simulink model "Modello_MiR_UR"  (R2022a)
settings: Solver=FixedStepAuto  StartTime=0.0  StopTime=time_s(end,1)  FixedStep=Sim.dt*10  RelTol=1e-3  EnableMultiTasking=on
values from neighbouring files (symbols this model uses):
  a = 0.250    (= 0.25)    [Modello_MiR_UR_script.m]    (also in Modello_MiR_2ruote_script.m; Modello_MiR_6ruote_script.m; Modello_MiR_6ruote_validato_script.m)
  a1 = 0.18265    [Modello_MiR_UR_script.m]    (also in UR_DHtable_e.m = 0; Modello_MiR_2ruote_script.m = deg2rad(5); Modello_MiR_6ruote_script.m = deg2rad(5); Modello_MiR_6ruote_validato_script.m)
  a2 = 0.40857    [Modello_MiR_UR_script.m]    (also in UR_DHtable_e.m = 612; Modello_MiR_2ruote_script.m = deg2rad(25); Modello_MiR_6ruote_script.m = deg2rad(25); Modello_MiR_6ruote_validato_script.m)
  Att_C1 = 0.01    [Modello_MiR_UR_script.m]    (also in Modello_MiR_6ruote_validato_script.m)
  Att_C2 = 0.01    [Modello_MiR_UR_script.m]    (also in Modello_MiR_6ruote_validato_script.m)
  Att_C5 = 0.01    [Modello_MiR_UR_script.m]    (also in Modello_MiR_6ruote_validato_script.m)
  Att_C6 = 0.01    [Modello_MiR_UR_script.m]    (also in Modello_MiR_6ruote_validato_script.m)
  b = 0.1875    [Modello_MiR_UR_script.m]    (also in Modello_MiR_2ruote_script.m; Modello_MiR_6ruote_script.m; Modello_MiR_6ruote_validato_script.m)
  b_caster = 0.07    [Modello_MiR_UR_script.m]    (also in Modello_MiR_2ruote_script.m; Modello_MiR_6ruote_script.m; Modello_MiR_6ruote_validato_script.m)
  bd = 0.205    [Modello_MiR_UR_script.m]    (also in Modello_MiR_2ruote_script.m; Modello_MiR_6ruote_script.m; Modello_MiR_6ruote_validato_script.m)
  F23MIR = @(u) (mv*9.801/4)-(mv*h*u(5)+(mv*9.801/4)*(2*a-b_caster*(cos(u(1))+cos(u(2)))))/(4*a-b_caster*(cos(u(1))+cos(u(2)))+b_caster*(cos(u(3))+cos(u(4))))    [Modello_MiR_UR_script.m]
  F23UR5 = @(u) (u(7)/4)-u(11)    [Modello_MiR_UR_script.m]
  F43MIR = @(u) (1/(2*bd))*(mv*u(6)*h+((mv*h*u(5)+(mv*9.801/4)*(2*a-b_caster*(cos(u(1))+cos(u(2)))))/(4*a-b_caster*(cos(u(1))+cos(u(2)))+b_caster*(cos(u(3))+cos(u(4)))))*(2*bd-b_caster*(sin(u(3))+sin(u(4))))+((mv*9.801/4)-(mv*h*u(5)+(mv*9.801/4)*(2*a-b_caster*(cos(u(1))+cos(u(2)))))/(4*a-b_caster*(cos(u(1))+cos(u(2)))+b_caster*(cos(u(3))+cos(u(4)))))*(2*bd-b_caster*(sin(u(1))+sin(u(2)))))    [Modello_MiR_UR_script.m]
  F43UR5 = @(u) (1/(2*bd))*(u(8) - u(6)*H +u(11)*(2*bd-b_caster*(sin(u(3))+sin(u(4))))+u(12)*(2*bd-b_caster*(sin(u(1))+sin(u(2)))))    [Modello_MiR_UR_script.m]
  F63MIR = @(u) (mv*h*u(5)+(mv*9.801/4)*(2*a-b_caster*(cos(u(1))+cos(u(2)))))/(4*a-b_caster*(cos(u(1))+cos(u(2)))+b_caster*(cos(u(3))+cos(u(4))))    [Modello_MiR_UR_script.m]
  F63UR5 = @(u)(-a*u(7)/2 -u(5)*H -u(9) +(u(7)/4)*(2*a-b_caster*(cos(u(1))+cos(u(2)))))/(4*a-b_caster*(cos(u(1))+cos(u(2)))+b_caster*(cos(u(3))+cos(u(4))))    [Modello_MiR_UR_script.m]
  f_c = 0.29564    [Modello_MiR_UR_script.m]    (also in Modello_MiR_6ruote_validato_script.m)
  f_d3 = 0.35846    [Modello_MiR_UR_script.m]    (also in Modello_MiR_6ruote_validato_script.m)
  f_d4 = 0.2333    [Modello_MiR_UR_script.m]    (also in Modello_MiR_6ruote_validato_script.m)
  fa_c = 0.27474    [Modello_MiR_UR_script.m]    (also in Modello_MiR_6ruote_validato_script.m)
  fa_d3 = 0.3694    [Modello_MiR_UR_script.m]    (also in Modello_MiR_6ruote_validato_script.m)
  fa_d4 = 0.28065    [Modello_MiR_UR_script.m]    (also in Modello_MiR_6ruote_validato_script.m)
  fm_fun = @(u) (u <= -am2 || u >= am2) * 0 + (u > -am2 && u <= -am1) * (- u* Mza/(am2 -am1) - Mza* am2/(am2 -am1)) +           + (u > -am1 && u <= am1) * (Mza * u / am1) + (u > am1 && u < am2) * (Mza * u /(am1 -am2) - Mza * am2 /(am1 - am2))    [Modello_MiR_UR_script.m]    (also in Modello_MiR_6ruote_script.m = @(u) (u <= -am2 | u >= am2)*0 + (u > -am2 && u <= -am1)*(- u; Modello_MiR_6ruote_validato_script.m)
  Hi = 1    [UR5e_data.m]
  Icw_1 = 1/2 * mcw * rc^2    (= 0.002004225735)    [Modello_MiR_UR_script.m]    (also in Modello_MiR_2ruote_script.m; Modello_MiR_6ruote_script.m; Modello_MiR_6ruote_validato_script.m)
  Icw_2 = 1/12 * mcw * ec^2 + 1/4 * mcw * rc^2    (= 0.00104098243873)    [Modello_MiR_UR_script.m]    (also in Modello_MiR_2ruote_script.m; Modello_MiR_6ruote_script.m; Modello_MiR_6ruote_validato_script.m)
  Idw_1 = 1/2 * mdw * rd^2    (= 0.00551836278784)    [Modello_MiR_UR_script.m]    (also in Modello_MiR_2ruote_script.m; Transfer_Function_Gol_Gcl.m = Inertia_vect(jj,1); Modello_MiR_6ruote_script.m; Modello_MiR_6ruote_validato_script.m)
  iMax = 20.7*1.1    (= 22.77)    [Modello_MiR_UR_script.m]    (also in Modello_MiR_2ruote_script.m; Modello_MiR_6ruote_script.m; Modello_MiR_6ruote_validato_script.m)
  Iv = mv * (l^2 + w^2)  / 12    (= 6.75343333333)    [Modello_MiR_UR_script.m]    (also in Modello_MiR_2ruote_script.m; Modello_MiR_6ruote_script.m; Modello_MiR_6ruote_validato_script.m = 8.95033333333)
  Kc = 0.15    [Modello_MiR_UR_script.m]    (also in Modello_MiR_2ruote_script.m; Modello_MiR_6ruote_script.m; Modello_MiR_6ruote_validato_script.m)
  Ki_i = 1    [Modello_MiR_UR_script.m]    (also in Modello_MiR_2ruote_script.m; Modello_MiR_6ruote_script.m; Modello_MiR_6ruote_validato_script.m)
  Ki_v = 1    [Modello_MiR_UR_script.m]    (also in Modello_MiR_2ruote_script.m; Modello_MiR_6ruote_script.m; Modello_MiR_6ruote_validato_script.m)
  kk = 0.00005    (= 5e-05)    [Modello_MiR_UR_script.m]    (also in Modello_MiR_2ruote_script.m; Modello_MiR_6ruote_script.m; Modello_MiR_6ruote_validato_script.m)
  Kp_i = 5    [Modello_MiR_UR_script.m]    (also in Modello_MiR_2ruote_script.m; Modello_MiR_6ruote_script.m; Modello_MiR_6ruote_validato_script.m)
  Kp_v = 5    [Modello_MiR_UR_script.m]    (also in Modello_MiR_2ruote_script.m; Modello_MiR_6ruote_script.m; Modello_MiR_6ruote_validato_script.m)
  kv = 1.5e-6    (= 1.5e-06)    [Modello_MiR_UR_script.m]    (also in Modello_MiR_2ruote_script.m; Modello_MiR_6ruote_script.m; Modello_MiR_6ruote_validato_script.m)
  L = R * tauE    (= 0.00181134822805)    [Modello_MiR_UR_script.m]    (also in Modello_MiR_2ruote_script.m; Modello_MiR_6ruote_script.m; Modello_MiR_6ruote_validato_script.m)
  mcw = rc^2 * pi * ec * rhopoliu + 1    (= 1.02616357632)    [Modello_MiR_UR_script.m]    (also in Modello_MiR_2ruote_script.m; Modello_MiR_6ruote_script.m; Modello_MiR_6ruote_validato_script.m)
  mv = 83    [Modello_MiR_UR_script.m]    (also in Modello_MiR_2ruote_script.m; Modello_MiR_6ruote_script.m; Modello_MiR_6ruote_validato_script.m = 110)
  Phi1_start = psi_mir(1,1)    [Modello_MiR_UR_script.m]    (also in Modello_MiR_6ruote_validato_script.m)
  Phi2_start = psi_mir(1,1)    [Modello_MiR_UR_script.m]    (also in Modello_MiR_6ruote_validato_script.m)
  Phi5_start = psi_mir(1,1)    [Modello_MiR_UR_script.m]    (also in Modello_MiR_6ruote_validato_script.m)
  Phi6_start = psi_mir(1,1)    [Modello_MiR_UR_script.m]    (also in Modello_MiR_6ruote_validato_script.m)
  Psi_start = psi_mir(1,1)    [Modello_MiR_UR_script.m]    (also in Modello_MiR_6ruote_script.m = 1.57079632679; Modello_MiR_6ruote_validato_script.m)
  q0 = [qset.q1.signals.values(1),qset.q2.signals.values(1),qset.q3.signals.values(1),qset.q4.signals.values(1),qset.q5.signals.values(1),qset.q6.signals.values(1)]    [UR5e_simmot.m]
  R = velMax * TorqueMax / (iMax)^2    (= 1.81134822805)    [Modello_MiR_UR_script.m]    (also in Modello_MiR_2ruote_script.m; Modello_MiR_6ruote_script.m; Modello_MiR_6ruote_validato_script.m)
  rap_rid = 10.167    [Modello_MiR_UR_script.m]    (also in Modello_MiR_2ruote_script.m; Modello_MiR_6ruote_script.m; Modello_MiR_6ruote_validato_script.m)
  rc = 0.125/2    (= 0.0625)    [Modello_MiR_UR_script.m]    (also in Modello_MiR_2ruote_script.m; Modello_MiR_6ruote_script.m; Modello_MiR_6ruote_validato_script.m)
  rd = 0.1    [Modello_MiR_UR_script.m]    (also in Modello_MiR_2ruote_script.m; Modello_MiR_6ruote_script.m; Modello_MiR_6ruote_validato_script.m)
  s = 1i*s    [Transfer_Function_Gol_Gcl.m]
  s1 = 0.18987    [Modello_MiR_UR_script.m]    (also in Modello_MiR_2ruote_script.m = 0.2; Modello_MiR_6ruote_script.m = 0.2; Modello_MiR_6ruote_validato_script.m)
  s2 = 0.99533    [Modello_MiR_UR_script.m]    (also in Modello_MiR_2ruote_script.m = 0.8; Modello_MiR_6ruote_script.m = 0.8; Modello_MiR_6ruote_validato_script.m)
  Sx = spline(x ,fl_fun(x),zx)    [Modello_MiR_6ruote_script.m]
  Sy = spline(x ,ft_fun(x),zy)    [Modello_MiR_6ruote_script.m]
  tau_i = 1/(2000*2*pi)    (= 7.95774715459e-05)    [UR5e_data.m]    (also in Transfer_Function_Gol_Gcl.m = Kp_i/Ki_i)
  VaMax = Kc * velMax    (= 41.2443991527)    [Modello_MiR_UR_script.m]    (also in Modello_MiR_2ruote_script.m; Modello_MiR_6ruote_script.m; Modello_MiR_6ruote_validato_script.m)
  X_start = traj(1,1)    [Modello_MiR_UR_script.m]    (also in Modello_MiR_2ruote_script.m = input('Inserire coordinata x iniziale'); Modello_MiR_6ruote_script.m = input('Inserire coordinata x iniziale'); Modello_MiR_6ruote_validato_script.m)
  Y_start = traj(1,2)    [Modello_MiR_UR_script.m]    (also in Modello_MiR_2ruote_script.m = input('Inserire coordinata y iniziale'); Modello_MiR_6ruote_script.m = input('Inserire coordinata y iniziale'); Modello_MiR_6ruote_validato_script.m)
undefined symbols (not defined in the file or in its folder): deg, Driver1, Driver2, Driver3, Driver4, Driver5, Driver6, Ground, J1, J2, J3, J4, J5, J6, kg, L1, L2, L3, L4, L5, L6, m, Motor, N, X, Y, z, Z
libraries: sm_lib x33, nesl_utility x30, slpidlib x10
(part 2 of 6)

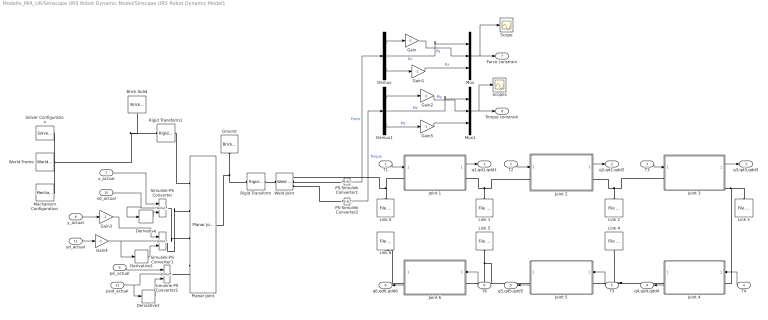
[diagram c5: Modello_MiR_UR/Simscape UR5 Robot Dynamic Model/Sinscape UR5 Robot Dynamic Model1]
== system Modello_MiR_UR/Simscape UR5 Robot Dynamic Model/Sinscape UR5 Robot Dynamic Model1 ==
  T1 : Inport
  T2 : Inport  Port=2
  T3 : Inport  Port=3
  T4 : Inport  Port=4
  T5 : Inport  Port=5
  T6 : Inport  Port=6
  x_actual : Inport  Port=7
  y_actual : Inport  Port=8
  psi_actual : Inport  Port=9
  xd_actual : Inport  Port=10
  yd_actual : Inport  Port=11
  psid_actual : Inport  Port=12
  Brick Solid : sm_lib/Body Elements/Brick Solid  GraphicAmbientColor=[0.15 0.15 0.15 1.0]  BasedOnType=Density  BrickDimensions=[100 100 1]  BrickDimensionUnits=m  CenterOfMass=[0 0 0]  CenterOfMassUnits=m  GraphicDiffuseColor=[0.5 0.5 0.5]  Density=1000  DensityUnits=kg/m^3  DoExposeReferenceFrame=on  GraphicEmissiveColor=[0.0 0.0 0.0 1.0]  ExportEntireGeometry=off  SerializedFrames=<Frames/>  MarkerShape=Sphere  MarkerSize=10  GraphicType=FromGeometry  InertiaType=CalculateFromGeometry  Mass=1  MassUnits=kg  MomentsOfInertia=[1 1 1]  MomentsOfInertiaUnits=kg*m^2  GraphicOpacity=1.0  ProductsOfInertia=[0 0 0]  ProductsOfInertiaUnits=kg*m^2  GraphicShininess=75  GraphicSpecularColor=[0.5 0.5 0.5 1.0]  GraphicVisPropType=SimpleVisualProperties
  Demux : Demux  Outputs=3
  Demux1 : Demux  Outputs=3
  Derivative : Derivative
  Derivative1 : Derivative
  Derivative2 : Derivative
  Gain{,1..5} (6 alike) : Gain  Gain=-1
  Ground : sm_lib/Body Elements/Brick Solid  GraphicAmbientColor=[0.15 0.15 0.15 1.0]  BasedOnType=Density  BrickDimensions=[Ground.l Ground.w Ground.h]  BrickDimensionUnits=m  CenterOfMass=[0 0 0]  CenterOfMassUnits=m  GraphicDiffuseColor=[1.0 1.0 1.0]  Density=1000  DensityUnits=kg/m^3  DoExposeReferenceFrame=on  GraphicEmissiveColor=[0.0 0.0 0.0 1.0]  ExportEntireGeometry=off  SerializedFrames=<Frames/>  MarkerShape=Sphere  MarkerSize=10  GraphicType=FromGeometry  InertiaType=CalculateFromGeometry  Mass=1  MassUnits=kg  MomentsOfInertia=[1 1 1]  MomentsOfInertiaUnits=kg*m^2  GraphicOpacity=1.0  ProductsOfInertia=[0 0 0]  ProductsOfInertiaUnits=kg*m^2  GraphicShininess=75  GraphicSpecularColor=[0.5 0.5 0.5 1.0]  GraphicVisPropType=SimpleVisualProperties
  Joint 1 : Subsystem
  Joint 2 : Subsystem
  Joint 3 : Subsystem
  Joint 4 : Subsystem
  Joint 5 : Subsystem
  Joint 6 : Subsystem
  Link 0 : sm_lib/Body Elements/File Solid  ExtGeomFileName=C:\Users\user\Desktop\Modello MiR-UR validato\GROUND.stp  UnitType=Custom  ExtGeomFileUnits=mm  StepReaderType=HEX  ExportConvexHullGeometry=off  InertiaType=Custom  Mass=1  MassUnits=kg  CenterOfMass=[0 0 0]  CenterOfMassUnits=m  MomentsOfInertia=[1 1 1]  MomentsOfInertiaUnits=kg*m^2  ProductsOfInertia=[0 0 0]  ProductsOfInertiaUnits=kg*m^2  BasedOnType=DensityFromFile  Density=1000  DensityUnits=kg/m^3  DoExposeReferenceFrame=on  SerializedFrames=<Frames/>  GraphicType=FromGeometry  MarkerShape=Sphere  MarkerSize=10  GraphicVisPropType=SimpleVisualProperties  GraphicDiffuseColor=[0.5 0.5 0.5]  GraphicSpecularColor=[0.5 0.5 0.5 1.0]  GraphicAmbientColor=[0.15 0.15 0.15 1.0]  GraphicEmissiveColor=[0.0 0.0 0.0 1.0]  GraphicShininess=75  GraphicOpacity=1.0
  Link 1 : sm_lib/Body Elements/File Solid  ExtGeomFileName=C:\Users\user\Desktop\Modello MiR-UR validato\UR5 old\LINK1.STEP  UnitType=Custom  ExtGeomFileUnits=mm  StepReaderType=HEX  ExportConvexHullGeometry=off  InertiaType=Custom  Mass=L1.Mass  MassUnits=kg  CenterOfMass=L1.CM  CenterOfMassUnits=m  MomentsOfInertia=L1.InertiaM  MomentsOfInertiaUnits=kg*m^2  ProductsOfInertia=L1.InertiaP  ProductsOfInertiaUnits=kg*m^2  BasedOnType=DensityFromFile  Density=1000  DensityUnits=kg/m^3  DoExposeReferenceFrame=on  SerializedFrames=<Frames/>  GraphicType=FromGeometry  MarkerShape=Sphere  MarkerSize=10  GraphicVisPropType=SimpleVisualProperties  GraphicDiffuseColor=[0.5 0.5 0.5]  GraphicSpecularColor=[0.5 0.5 0.5 1.0]  GraphicAmbientColor=[0.15 0.15 0.15 1.0]  GraphicEmissiveColor=[0.0 0.0 0.0 1.0]  GraphicShininess=75  GraphicOpacity=1.0
  Link 2 : sm_lib/Body Elements/File Solid  ExtGeomFileName=C:\Users\user\Desktop\Modello MiR-UR validato\UR5 old\LINK2.STEP  UnitType=Custom  ExtGeomFileUnits=mm  StepReaderType=HEX  ExportConvexHullGeometry=off  InertiaType=Custom  Mass=L2.Mass  MassUnits=kg  CenterOfMass=L2.CM  CenterOfMassUnits=m  MomentsOfInertia=L2.InertiaM  MomentsOfInertiaUnits=kg*m^2  ProductsOfInertia=L2.InertiaP  ProductsOfInertiaUnits=kg*m^2  BasedOnType=DensityFromFile  Density=1000  DensityUnits=kg/m^3  DoExposeReferenceFrame=on  SerializedFrames=<Frames/>  GraphicType=FromGeometry  MarkerShape=Sphere  MarkerSize=10  GraphicVisPropType=SimpleVisualProperties  GraphicDiffuseColor=[0.5 0.5 0.5]  GraphicSpecularColor=[0.5 0.5 0.5 1.0]  GraphicAmbientColor=[0.15 0.15 0.15 1.0]  GraphicEmissiveColor=[0.0 0.0 0.0 1.0]  GraphicShininess=75  GraphicOpacity=1.0
  Link 3 : sm_lib/Body Elements/File Solid  ExtGeomFileName=C:\Users\user\Desktop\Modello MiR-UR validato\UR5 old\LINK3.STEP  UnitType=Custom  ExtGeomFileUnits=mm  StepReaderType=HEX  ExportConvexHullGeometry=off  InertiaType=Custom  Mass=L3.Mass  MassUnits=kg  CenterOfMass=L3.CM  CenterOfMassUnits=m  MomentsOfInertia=L3.InertiaM  MomentsOfInertiaUnits=kg*m^2  ProductsOfInertia=L3.InertiaP  ProductsOfInertiaUnits=kg*m^2  BasedOnType=DensityFromFile  Density=1000  DensityUnits=kg/m^3  DoExposeReferenceFrame=on  SerializedFrames=<Frames/>  GraphicType=FromGeometry  MarkerShape=Sphere  MarkerSize=10  GraphicVisPropType=SimpleVisualProperties  GraphicDiffuseColor=[0.5 0.5 0.5]  GraphicSpecularColor=[0.5 0.5 0.5 1.0]  GraphicAmbientColor=[0.15 0.15 0.15 1.0]  GraphicEmissiveColor=[0.0 0.0 0.0 1.0]  GraphicShininess=75  GraphicOpacity=1.0
  Link 4 : sm_lib/Body Elements/File Solid  ExtGeomFileName=C:\Users\user\Desktop\Modello MiR-UR validato\UR5 old\LINK4.STEP  UnitType=Custom  ExtGeomFileUnits=mm  StepReaderType=HEX  ExportConvexHullGeometry=off  InertiaType=Custom  Mass=L4.Mass  MassUnits=kg  CenterOfMass=L4.CM  CenterOfMassUnits=m  MomentsOfInertia=L4.InertiaM  MomentsOfInertiaUnits=kg*m^2  ProductsOfInertia=L4.InertiaP  ProductsOfInertiaUnits=kg*m^2  BasedOnType=DensityFromFile  Density=1000  DensityUnits=kg/m^3  DoExposeReferenceFrame=on  SerializedFrames=<Frames/>  GraphicType=FromGeometry  MarkerShape=Sphere  MarkerSize=10  GraphicVisPropType=SimpleVisualProperties  GraphicDiffuseColor=[0.5 0.5 0.5]  GraphicSpecularColor=[0.5 0.5 0.5 1.0]  GraphicAmbientColor=[0.15 0.15 0.15 1.0]  GraphicEmissiveColor=[0.0 0.0 0.0 1.0]  GraphicShininess=75  GraphicOpacity=1.0
  Link 5 : sm_lib/Body Elements/File Solid  ExtGeomFileName=C:\Users\user\Desktop\Modello MiR-UR validato\UR5 old\LINK5.STEP  UnitType=Custom  ExtGeomFileUnits=mm  StepReaderType=HEX  ExportConvexHullGeometry=off  InertiaType=Custom  Mass=L5.Mass  MassUnits=kg  CenterOfMass=L5.CM  CenterOfMassUnits=m  MomentsOfInertia=L5.InertiaM  MomentsOfInertiaUnits=kg*m^2  ProductsOfInertia=L5.InertiaP  ProductsOfInertiaUnits=kg*m^2  BasedOnType=DensityFromFile  Density=1000  DensityUnits=kg/m^3  DoExposeReferenceFrame=on  SerializedFrames=<Frames/>  GraphicType=FromGeometry  MarkerShape=Sphere  MarkerSize=10  GraphicVisPropType=SimpleVisualProperties  GraphicDiffuseColor=[0.5 0.5 0.5]  GraphicSpecularColor=[0.5 0.5 0.5 1.0]  GraphicAmbientColor=[0.15 0.15 0.15 1.0]  GraphicEmissiveColor=[0.0 0.0 0.0 1.0]  GraphicShininess=75  GraphicOpacity=1.0
  Link 6 : sm_lib/Body Elements/File Solid  ExtGeomFileName=C:\Users\user\Desktop\Modello MiR-UR validato\UR5 old\LINK6.STEP  UnitType=Custom  ExtGeomFileUnits=mm  StepReaderType=HEX  ExportConvexHullGeometry=off  InertiaType=Custom  Mass=L6.Mass  MassUnits=kg  CenterOfMass=L6.CM  CenterOfMassUnits=m  MomentsOfInertia=L6.InertiaM  MomentsOfInertiaUnits=kg*m^2  ProductsOfInertia=L6.InertiaP  ProductsOfInertiaUnits=kg*m^2  BasedOnType=DensityFromFile  Density=1000  DensityUnits=kg/m^3  DoExposeReferenceFrame=on  SerializedFrames=<Frames/>  GraphicType=FromGeometry  MarkerShape=Sphere  MarkerSize=10  GraphicVisPropType=SimpleVisualProperties  GraphicDiffuseColor=[0.5 0.5 0.5]  GraphicSpecularColor=[0.5 0.5 0.5 1.0]  GraphicAmbientColor=[0.15 0.15 0.15 1.0]  GraphicEmissiveColor=[0.0 0.0 0.0 1.0]  GraphicShininess=75  GraphicOpacity=1.0
  Mechanism Configuration : sm_lib/Utilities/Mechanism Configuration  UniformGravity=Constant  GravityVector=[0 0 -9.80665]  GravityUnits=m/s^2  LinearizationDelta=0.001  JointModeTransitionNonlinearIterations=2
  Mux : Mux  Inputs=3
  Mux1 : Mux  Inputs=3
  PS-Simulink Converter1 : nesl_utility/PS-Simulink Converter  PhysicalDomain=network_engine_domain  SubClassName=ps_output  LeftPortType=input  RightPortType=output  PseudoPeriodic=off  Frequencies=[]  VectorFormat=1-D array  Unit=1  AffineConversion=off
  PS-Simulink Converter2 : nesl_utility/PS-Simulink Converter  PhysicalDomain=network_engine_domain  SubClassName=ps_output  LeftPortType=input  RightPortType=output  PseudoPeriodic=off  Frequencies=[]  VectorFormat=1-D array  Unit=1  AffineConversion=off
  Planar Joint : sm_lib/Joints/Planar Joint  JointMode=Normal  SenseConstraintForce=off  SenseConstraintForceX=off  SenseConstraintForceY=off  SenseConstraintForceZ=off  SenseConstraintTorque=off  SenseConstraintTorqueX=off  SenseConstraintTorqueY=off  SenseConstraintTorqueZ=off  SenseTotalForce=off  SenseTotalForceX=off  SenseTotalForceY=off  SenseTotalForceZ=off  SenseTotalTorque=off  SenseTotalTorqueX=off  SenseTotalTorqueY=off  SenseTotalTorqueZ=off  CompositeWrenchDir=FollowerOnBase  CompositeWrenchFrame=BaseFrame  PxEquilibriumPosition=0  PxEquilibriumPositionUnits=m  PxSpringStiffness=0  PxSpringStiffnessUnits=N/m  PxDampingCoefficient=0  PxDampingCoefficientUnits=N/(m/s)  PxTorqueActuationMode=ComputedTorque  PxMotionActuationMode=InputMotion  PxSensePosition=off  PxSenseVelocity=off  PxSenseAcceleration=off  PxSenseTorqueForce=off  PxSenseLowerLimitTorqueForce=off  PxSenseUpperLimitTorqueForce=off  PxLowerLimitSpecify=off  PxLowerLimitBound=-1  PxLowerLimitBoundUnits=m  PxLowerLimitStiffness=1e6  PxLowerLimitStiffnessUnits=N/m  PxLowerLimitDamping=1e3  PxLowerLimitDampingUnits=N/(m/s)  PxLowerLimitTransitionRegionWidth=1e-4  PxLowerLimitTransitionRegionWidthUnits=m  PxUpperLimitSpecify=off  PxUpperLimitBound=1  PxUpperLimitBoundUnits=m  PxUpperLimitStiffness=1e6  PxUpperLimitStiffnessUnits=N/m  PxUpperLimitDamping=1e3  PxUpperLimitDampingUnits=N/(m/s)  PxUpperLimitTransitionRegionWidth=1e-4  PxUpperLimitTransitionRegionWidthUnits=m  PxPositionTargetSpecify=on  PxPositionTargetPriority=High  PxPositionTargetValue=0  PxPositionTargetValueUnits=m  PxVelocityTargetSpecify=on  PxVelocityTargetPriority=High  PxVelocityTargetValue=0  PxVelocityTargetValueUnits=m/s  PyEquilibriumPosition=0  PyEquilibriumPositionUnits=m  PySpringStiffness=0  PySpringStiffnessUnits=N/m  PyDampingCoefficient=0  PyDampingCoefficientUnits=N/(m/s)  PyTorqueActuationMode=ComputedTorque  PyMotionActuationMode=InputMotion  PySensePosition=off  PySenseVelocity=off  PySenseAcceleration=off  PySenseTorqueForce=off  PySenseLowerLimitTorqueForce=off  PySenseUpperLimitTorqueForce=off  PyLowerLimitSpecify=off  PyLowerLimitBound=-1  PyLowerLimitBoundUnits=m  PyLowerLimitStiffness=1e6  PyLowerLimitStiffnessUnits=N/m  PyLowerLimitDamping=1e3  PyLowerLimitDampingUnits=N/(m/s)  PyLowerLimitTransitionRegionWidth=1e-4  PyLowerLimitTransitionRegionWidthUnits=m  PyUpperLimitSpecify=off  PyUpperLimitBound=1  PyUpperLimitBoundUnits=m  PyUpperLimitStiffness=1e6  PyUpperLimitStiffnessUnits=N/m  PyUpperLimitDamping=1e3  PyUpperLimitDampingUnits=N/(m/s)  PyUpperLimitTransitionRegionWidth=1e-4  PyUpperLimitTransitionRegionWidthUnits=m  PyPositionTargetSpecify=on  PyPositionTargetPriority=High  PyPositionTargetValue=0  PyPositionTargetValueUnits=m  PyVelocityTargetSpecify=on  PyVelocityTargetPriority=High  PyVelocityTargetValue=0  PyVelocityTargetValueUnits=m/s  RzEquilibriumPosition=0  RzEquilibriumPositionUnits=deg  RzSpringStiffness=0  RzSpringStiffnessUnits=N*m/deg  RzDampingCoefficient=0  RzDampingCoefficientUnits=N*m/(deg/s)  RzTorqueActuationMode=ComputedTorque  RzMotionActuationMode=InputMotion  RzSensePosition=off  RzSenseVelocity=off  RzSenseAcceleration=off  RzSenseTorqueForce=off  RzSenseLowerLimitTorqueForce=off  RzSenseUpperLimitTorqueForce=off  RzLowerLimitSpecify=off  RzLowerLimitBound=-90  RzLowerLimitBoundUnits=deg  RzLowerLimitStiffness=1e4  RzLowerLimitStiffnessUnits=N*m/deg  RzLowerLimitDamping=10  RzLowerLimitDampingUnits=N*m/(deg/s)  RzLowerLimitTransitionRegionWidth=0.1  RzLowerLimitTransitionRegionWidthUnits=deg  RzUpperLimitSpecify=off  RzUpperLimitBound=90  RzUpperLimitBoundUnits=deg  RzUpperLimitStiffness=1e4  RzUpperLimitStiffnessUnits=N*m/deg  RzUpperLimitDamping=10  RzUpperLimitDampingUnits=N*m/(deg/s)  RzUpperLimitTransitionRegionWidth=0.1  RzUpperLimitTransitionRegionWidthUnits=deg  RzPositionTargetSpecify=on  RzPositionTargetPriority=High  RzPositionTargetValue=pi/2  RzPositionTargetValueUnits=deg  RzVelocityTargetSpecify=on  RzVelocityTargetPriority=High  RzVelocityTargetValue=0  RzVelocityTargetValueUnits=deg/s
  Rigid Transform : sm_lib/Frames and Transforms/Rigid Transform  TranslationMethod=Cartesian  TranslationStandardOffset=0  TranslationLengthUnit=m  TranslationStandardAxis=+Z  TranslationCartesianOffset=[0 0 (Ground.h/2)]  TranslationROffset=0  TranslationROffsetUnits=m  TranslationZOffset=0  TranslationZOffsetUnits=m  TranslationThetaOffset=0  TranslationThetaOffsetUnits=deg  RotationMethod=RotationSequence  RotationAngleUnits=deg  RotationStandardAxis=+Z  RotationAngle=0.0  RotationArbitraryAxis=[0 0 1]  FollAlignAxisA=+X  BaseAlignAxisA=+Y  FollAlignAxisB=+Y  BaseAlignAxisB=+Z  RotationSequenceAxes=BaseAxes  RotationSequence=XYZ  RotationSequenceAngles=[0 0 -90]  RotationSequenceAnglesUnits=deg  RotationMatrix=[1 0 0; 0 1 0; 0 0 1]
  Rigid Transform1 : sm_lib/Frames and Transforms/Rigid Transform  TranslationMethod=Cartesian  TranslationStandardOffset=0  TranslationLengthUnit=m  TranslationStandardAxis=+Z  TranslationCartesianOffset=[0 0 0.5]  TranslationROffset=0  TranslationROffsetUnits=m  TranslationZOffset=0  TranslationZOffsetUnits=m  TranslationThetaOffset=0  TranslationThetaOffsetUnits=deg  RotationMethod=RotationSequence  RotationAngleUnits=deg  RotationStandardAxis=+Z  RotationAngle=0.0  RotationArbitraryAxis=[0 0 1]  FollAlignAxisA=+X  BaseAlignAxisA=+Y  FollAlignAxisB=+Y  BaseAlignAxisB=+Z  RotationSequenceAxes=BaseAxes  RotationSequence=XYZ  RotationSequenceAngles=[0 0 -90]  RotationSequenceAnglesUnits=deg  RotationMatrix=[1 0 0; 0 1 0; 0 0 1]
  Scope : Scope
  Scope1 : Scope
  Simulink-PS Converter : nesl_utility/Simulink-PS Converter  PhysicalDomain=network_engine_domain  SubClassName=ps_input  LeftPortType=input  RightPortType=output  PseudoPeriodic=off  Frequencies=[]  NoiseDistribution=none  NoiseParameters=[]  Unit=1  AffineConversion=off  FilteringAndDerivatives=provide  SimscapeFilterOrder=1  InputFilterTimeConstant=0.001  UdotUserProvided=2
  Simulink-PS Converter1 : nesl_utility/Simulink-PS Converter  PhysicalDomain=network_engine_domain  SubClassName=ps_input  LeftPortType=input  RightPortType=output  PseudoPeriodic=off  Frequencies=[]  NoiseDistribution=none  NoiseParameters=[]  Unit=1  AffineConversion=off  FilteringAndDerivatives=provide  SimscapeFilterOrder=1  InputFilterTimeConstant=0.001  UdotUserProvided=2
  Simulink-PS Converter2 : nesl_utility/Simulink-PS Converter  PhysicalDomain=network_engine_domain  SubClassName=ps_input  LeftPortType=input  RightPortType=output  PseudoPeriodic=off  Frequencies=[]  NoiseDistribution=none  NoiseParameters=[]  Unit=1  AffineConversion=off  FilteringAndDerivatives=provide  SimscapeFilterOrder=1  InputFilterTimeConstant=0.001  UdotUserProvided=2
  Solver Configuration : nesl_utility/Solver Configuration  PhysicalDomain=network_engine_domain  SubClassName=solver  LeftPortType=input  RightPortType=generic  Tones=[]  Harmonics=[]  SimulateNoise=off  Profile=off  UseLocalSampling=off  EnableSwitchedLinearOptims=on  FrequencyDomain=off  UseCCode=off  RelTol=0.001  AbsTol=1e-06  MinStep=1e-09  ToWorkspace=off  RevertToSquareIcSolve=off  NumHomotopyIterations=100  PhasorMode=off  PhasorModeNumHarmonics=1  IndexReductionMethod=DerivativeReplacement  DoDC=off  ResidualTolerance=1e-09  UseLocalSolver=off  LocalSolverChoice=NE_BACKWARD_EULER_ADVANCER  LocalSolverSampleTime=0.001  DoFixedCost=off  MaxNonlinIter=3  MaxModeIter=2  ComputeImpulses=off  ImpulseIterations=2  LinearAlgebra=Sparse  LinearAlgebraNumThread=0  EquationFormulation=NE_TIME_EF  DelaysMemoryBudget=1024  AutomaticFiltering=on  FilteringTimeConstant=0.001  PartitionStorageMethod=AS_NEEDED  PartitionMemoryBudget=1024  PartitionMethod=FAST
  Weld Joint : sm_lib/Joints/Weld Joint  JointMode=Normal  SenseConstraintForce=on  SenseConstraintForceX=off  SenseConstraintForceY=off  SenseConstraintForceZ=off  SenseConstraintTorque=on  SenseConstraintTorqueX=off  SenseConstraintTorqueY=off  SenseConstraintTorqueZ=off  SenseTotalForce=off  SenseTotalForceX=off  SenseTotalForceY=off  SenseTotalForceZ=off  SenseTotalTorque=off  SenseTotalTorqueX=off  SenseTotalTorqueY=off  SenseTotalTorqueZ=off  CompositeWrenchDir=FollowerOnBase  CompositeWrenchFrame=BaseFrame
  World Frame : sm_lib/Frames and Transforms/World Frame
  q1,qd1,qdd1 : Outport
  q2,qd2,qdd2 : Outport  Port=2
  q3,qd3,qdd3 : Outport  Port=3
  q4,qd4,qdd4 : Outport  Port=4
  q5,qd5,qdd5 : Outport  Port=5
  q6,qd6,qdd6 : Outport  Port=6
  Force constrain : Outport  Port=7
  Torque constrain : Outport  Port=8
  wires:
  T1/1 -> Joint 1/1(T1)
  T2/1 -> Joint 2/1(T2)
  Joint 2/1(q2,qd2,qdd2) -> q2,qd2,qdd2/1
  Joint 3/1(q3,qd3,qdd3) -> q3,qd3,qdd3/1
  Joint 4/1(q4,qd4,qdd4) -> q4,qd4,qdd4/1
  Joint 5/1(q5,qd5,qdd5) -> q5,qd5,qdd5/1
  Joint 6/1(q6,qd6,qdd6) -> q6,qd6,qdd6/1
  T3/1 -> Joint 3/1(T3)
  T4/1 -> Joint 4/1(T4)
  T5/1 -> Joint 5/1(T5)
  T6/1 -> Joint 6/1(T6)
  Joint 1/1(q1,qd1,qdd1) -> q1,qd1,qdd1/1
  y_actual/1 -> Gain3/1
  psi_actual/1 -> Simulink-PS Converter2/1
  yd_actual/1 -> Gain4/1
  psid_actual/1 -> Derivative2/1, Simulink-PS Converter2/2
  Derivative/1 -> Simulink-PS Converter/3
  Derivative1/1 -> Simulink-PS Converter1/3
  Derivative2/1 -> Simulink-PS Converter2/3
  PS-Simulink Converter1/1 -> Demux/1  "Force"
  Demux/1 -> Gain/1
  Demux/3 -> Gain1/1
  Gain1/1 -> Mux/3  "Rz"
  Mux/1 -> Scope/1, Force constrain/1
  Mux1/1 -> Scope1/1, Torque constrain/1
  Demux1/2 -> Mux1/1  "Mx"
  Demux1/1 -> Gain2/1
  Gain2/1 -> Mux1/2  "My"
  PS-Simulink Converter2/1 -> Demux1/1  "Torque"
  x_actual/1 -> Simulink-PS Converter/1
  xd_actual/1 -> Derivative/1, Simulink-PS Converter/2
  Gain3/1 -> Simulink-PS Converter1/1
  Gain4/1 -> Derivative1/1, Simulink-PS Converter1/2
  Gain/1 -> Mux/2  "Ry"
  Demux/2 -> Mux/1  "Rx"
  Demux1/3 -> Gain5/1  "Mz"
  Gain5/1 -> Mux1/3
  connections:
  Weld Joint/LConn1 -- Rigid Transform/RConn1
  Joint 4/RConn1 -- Link 4/RConn1 -- Joint 5/LConn1
  Link 2/RConn1 -- Joint 2/RConn1 -- Joint 3/LConn1
  Link 1/RConn1 -- Joint 1/RConn1 -- Joint 2/LConn1
  Link 3/RConn1 -- Joint 3/RConn1 -- Joint 4/LConn1
  Joint 6/RConn1 -- Link 6/RConn1
  Link 5/RConn1 -- Joint 5/RConn1 -- Joint 6/LConn1
  Link 0/RConn1 -- Weld Joint/RConn1 -- Joint 1/LConn1
  PS-Simulink Converter1/LConn1 -- Weld Joint/RConn2
  PS-Simulink Converter2/LConn1 -- Weld Joint/RConn3
  Ground/RConn1 -- Planar Joint/RConn1 -- Rigid Transform/LConn1
  Rigid Transform1/RConn1 -- Planar Joint/LConn1
  Mechanism Configuration/RConn1 -- World Frame/RConn1 -- Brick Solid/RConn1 -- Rigid Transform1/LConn1 -- Solver Configuration/RConn1
  Planar Joint/LConn4 -- Simulink-PS Converter2/RConn1
  Simulink-PS Converter/RConn1 -- Planar Joint/LConn3
  Simulink-PS Converter1/RConn1 -- Planar Joint/LConn2

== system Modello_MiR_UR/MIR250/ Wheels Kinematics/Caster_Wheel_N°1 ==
  xd_From1 : Inport
  yd_From1 : Inport  Port=2
  Psid_From1 : Inport  Port=3
  Psi_From1 : Inport  Port=4
  Delta_From1 : Inport  Port=5
  Deltad_From1 : Inport  Port=6
  Interpreted MATLAB Function : MATLABFcn  MATLABFcn=(u(1)^2+u(2)^2)^0.5
  Interpreted MATLAB Function2 : MATLABFcn  MATLABFcn=asin(u(2)/((u(1)^2+u(2)^2)^0.5+(1/cccc)*((u(1)^2+u(2)^2)==0)))
  Mux : Mux  Inputs=6
  Mux1 : Mux  Inputs=2
  xd_ruota1 : MATLABFcn  MATLABFcn=(u(6)+u(3))*b_caster*sin(u(5))+u(1)-u(3)*b
  yd_ruota1 : MATLABFcn  MATLABFcn=-(u(6)+u(3))*b_caster*cos(u(5))+u(2)+u(3)*a
  vx_ruota1 : Outport
  gamma1 : Outport  Port=2
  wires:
  Mux/1 -> xd_ruota1/1, yd_ruota1/1
  Mux1/1 -> Interpreted MATLAB Function/1, Interpreted MATLAB Function2/1
  yd_ruota1/1 -> Mux1/2  "yd_ruota1"
  yd_From1/1 -> Mux/2
  xd_ruota1/1 -> Mux1/1  "xd_ruota1"
  xd_From1/1 -> Mux/1
  Psid_From1/1 -> Mux/3
  Delta_From1/1 -> Mux/5
  Psi_From1/1 -> Mux/4
  Deltad_From1/1 -> Mux/6
  Interpreted MATLAB Function2/1 -> gamma1/1  "gamma1"
  Interpreted MATLAB Function/1 -> vx_ruota1/1  "vx_ruota1"

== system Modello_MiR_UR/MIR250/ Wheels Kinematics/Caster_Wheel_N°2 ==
  xd_From1 : Inport
  yd_From1 : Inport  Port=2
  Psid_From1 : Inport  Port=3
  Psi_From1 : Inport  Port=4
  Delta_From2 : Inport  Port=5
  Deltad_From2 : Inport  Port=6
  Interpreted MATLAB Function : MATLABFcn  MATLABFcn=(u(1)^2+u(2)^2)^0.5
  Interpreted MATLAB Function2 : MATLABFcn  MATLABFcn=asin(u(2)/((u(1)^2+u(2)^2)^0.5+(1/cccc)*((u(1)^2+u(2)^2)==0)))
  Mux : Mux  Inputs=6
  Mux1 : Mux  Inputs=2
  xd_ruota2 : MATLABFcn  MATLABFcn=(u(6)+u(3))*b_caster*sin(u(5))+u(1)+u(3)*b
  yd_ruota2 : MATLABFcn  MATLABFcn=-(u(6)+u(3))*b_caster*cos(u(5))+u(2)+u(3)*a
  vx_ruota2 : Outport
  gamma2 : Outport  Port=2
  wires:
  Mux/1 -> xd_ruota2/1, yd_ruota2/1
  Mux1/1 -> Interpreted MATLAB Function/1, Interpreted MATLAB Function2/1
  yd_ruota2/1 -> Mux1/2  "yd_ruota2"
  yd_From1/1 -> Mux/2
  xd_ruota2/1 -> Mux1/1  "xd_ruota2"
  xd_From1/1 -> Mux/1
  Psid_From1/1 -> Mux/3
  Delta_From2/1 -> Mux/5
  Psi_From1/1 -> Mux/4
  Deltad_From2/1 -> Mux/6
  Interpreted MATLAB Function2/1 -> gamma2/1  "gamma2"
  Interpreted MATLAB Function/1 -> vx_ruota2/1  "vx_ruota2"

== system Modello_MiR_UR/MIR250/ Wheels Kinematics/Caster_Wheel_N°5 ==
  xd_From1 : Inport
  yd_From1 : Inport  Port=2
  Psid_From1 : Inport  Port=3
  Psi_From1 : Inport  Port=4
  Delta_From5 : Inport  Port=5
  Deltad_From5 : Inport  Port=6
  Interpreted MATLAB Function : MATLABFcn  MATLABFcn=(u(1)^2+u(2)^2)^0.5
  Interpreted MATLAB Function2 : MATLABFcn  MATLABFcn=asin(u(2)/((u(1)^2+u(2)^2)^0.5+(1/cccc)*((u(1)^2+u(2)^2)==0)))
  Mux : Mux  Inputs=6
  Mux1 : Mux  Inputs=2
  xd_ruota5 : MATLABFcn  MATLABFcn=(u(6)+u(3))*b_caster*sin(u(5))+u(1)-u(3)*b
  yd_ruota5 : MATLABFcn  MATLABFcn=-(u(6)+u(3))*b_caster*cos(u(5))+u(2)-u(3)*a
  vx_ruota5 : Outport
  gamma5 : Outport  Port=2
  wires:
  Mux/1 -> xd_ruota5/1, yd_ruota5/1
  Mux1/1 -> Interpreted MATLAB Function/1, Interpreted MATLAB Function2/1
  yd_ruota5/1 -> Mux1/2  "yd_ruota5"
  yd_From1/1 -> Mux/2
  xd_ruota5/1 -> Mux1/1  "xd_ruota5"
  xd_From1/1 -> Mux/1
  Psid_From1/1 -> Mux/3
  Delta_From5/1 -> Mux/5
  Psi_From1/1 -> Mux/4
  Deltad_From5/1 -> Mux/6
  Interpreted MATLAB Function2/1 -> gamma5/1  "gamma5"
  Interpreted MATLAB Function/1 -> vx_ruota5/1  "v_ruota5"

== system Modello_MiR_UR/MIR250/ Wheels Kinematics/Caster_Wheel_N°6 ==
  xd_From1 : Inport
  yd_From1 : Inport  Port=2
  Psid_From1 : Inport  Port=3
  Psi_From1 : Inport  Port=4
  Delta_From6 : Inport  Port=5
  Deltad_From6 : Inport  Port=6
  Interpreted MATLAB Function : MATLABFcn  MATLABFcn=(u(1)^2+u(2)^2)^0.5
  Interpreted MATLAB Function2 : MATLABFcn  MATLABFcn=asin(u(2)/((u(1)^2+u(2)^2)^0.5+(1/cccc)*((u(1)^2+u(2)^2)==0)))
  Mux : Mux  Inputs=6
  Mux1 : Mux  Inputs=2
  xd_ruota6 : MATLABFcn  MATLABFcn=(u(6)+u(3))*b_caster*sin(u(5))+u(1)+u(3)*b
  yd_ruota6 : MATLABFcn  MATLABFcn=-(u(6)+u(3))*b_caster*cos(u(5))+u(2)-u(3)*a
  vx_ruota6 : Outport
  gamma6 : Outport  Port=2
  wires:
  Mux/1 -> xd_ruota6/1, yd_ruota6/1
  Mux1/1 -> Interpreted MATLAB Function/1, Interpreted MATLAB Function2/1
  yd_ruota6/1 -> Mux1/2  "yd_ruota6"
  yd_From1/1 -> Mux/2
  xd_ruota6/1 -> Mux1/1  "xd_ruota6"
  xd_From1/1 -> Mux/1
  Psid_From1/1 -> Mux/3
  Delta_From6/1 -> Mux/5
  Psi_From1/1 -> Mux/4
  Deltad_From6/1 -> Mux/6
  Interpreted MATLAB Function2/1 -> gamma6/1  "gamma6"
  Interpreted MATLAB Function/1 -> vx_ruota6/1  "v_ruota6"

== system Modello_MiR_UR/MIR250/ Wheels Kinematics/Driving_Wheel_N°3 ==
  xd_From1 : Inport
  yd_From1 : Inport  Port=2
  Psid_From1 : Inport  Port=3
  Interpreted MATLAB Function : MATLABFcn  MATLABFcn=u(1) - u(3)*bd
  Interpreted MATLAB Function1 : MATLABFcn  MATLABFcn=u(2)
  Interpreted MATLAB Function3 : MATLABFcn  MATLABFcn=asin(u(2)/((u(1)^2+u(2)^2)^0.5+(1/cccc)*((u(1)^2+u(2)^2)==0)))
  Mux : Mux  Inputs=3
  Mux1 : Mux  Inputs=2
  Scope1 : Scope
  vx_ruota3 : Outport
  gamma3 : Outport  Port=2
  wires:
  yd_From1/1 -> Mux/2
  xd_From1/1 -> Mux/1
  Psid_From1/1 -> Mux/3
  Mux/1 -> Interpreted MATLAB Function1/1, Interpreted MATLAB Function/1
  Interpreted MATLAB Function1/1 -> Mux1/2  "yd_ruota3"
  Interpreted MATLAB Function/1 -> vx_ruota3/1, Mux1/1  "xd_ruota3"
  Interpreted MATLAB Function3/1 -> gamma3/1  "gamma3"
  Mux1/1 -> Scope1/1, Interpreted MATLAB Function3/1

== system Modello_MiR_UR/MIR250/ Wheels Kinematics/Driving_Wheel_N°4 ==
  xd_From1 : Inport
  yd_From1 : Inport  Port=2
  Psid_From1 : Inport  Port=3
  Interpreted MATLAB Function : MATLABFcn  MATLABFcn=u(1) + u(3)*bd
  Interpreted MATLAB Function1 : MATLABFcn  MATLABFcn=u(2)
  Interpreted MATLAB Function3 : MATLABFcn  MATLABFcn=asin(u(2)/((u(1)^2+u(2)^2)^0.5+(1/cccc)*((u(1)^2+u(2)^2)==0)))
  Mux : Mux  Inputs=3
  Mux1 : Mux  Inputs=2
  Scope : Scope
  vx_ruota4 : Outport
  gamma4 : Outport  Port=2
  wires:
  yd_From1/1 -> Mux/2
  xd_From1/1 -> Mux/1
  Psid_From1/1 -> Mux/3
  Mux/1 -> Interpreted MATLAB Function1/1, Interpreted MATLAB Function/1
  Interpreted MATLAB Function1/1 -> Mux1/2  "yd_ruota4"
  Interpreted MATLAB Function/1 -> vx_ruota4/1, Mux1/1, Scope/1  "xd_ruota4"
  Mux1/1 -> Interpreted MATLAB Function3/1
  Interpreted MATLAB Function3/1 -> gamma4/1  "gamma4"

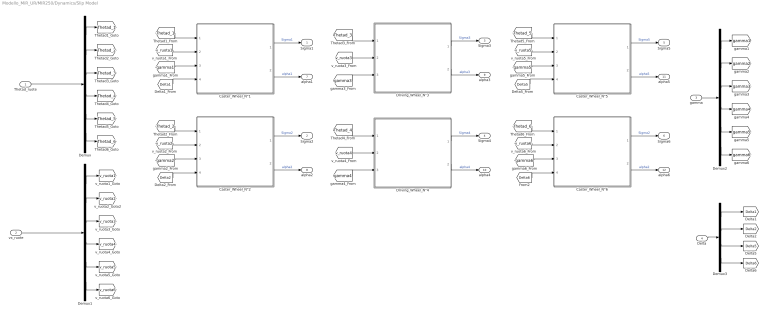
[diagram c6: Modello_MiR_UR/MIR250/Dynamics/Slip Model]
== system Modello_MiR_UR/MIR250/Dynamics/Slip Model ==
  Thetad_ruote : Inport
  vx_ruote : Inport  Port=2
  gamma : Inport  Port=3
  Delta : Inport  Port=4
  Caster_Wheel_N°1 : Subsystem
  Caster_Wheel_N°2 : Subsystem
  Caster_Wheel_N°5 : Subsystem
  Caster_Wheel_N°6 : Subsystem
  Demux : Demux  Outputs=6
  Demux1 : Demux  Outputs=6
  Demux2 : Demux  Outputs=6
  Demux3 : Demux
  Driving_Wheel_N°3 : Subsystem
  Driving_Wheel_N°4 : Subsystem
  Sigma1 : Outport
  Sigma2 : Outport  Port=2
  Sigma3 : Outport  Port=3
  Sigma4 : Outport  Port=4
  Sigma5 : Outport  Port=5
  Sigma6 : Outport  Port=6
  alpha1 : Outport  Port=7
  alpha2 : Outport  Port=8
  alpha3 : Outport  Port=9
  alpha4 : Outport  Port=10
  alpha5 : Outport  Port=11
  alpha6 : Outport  Port=12
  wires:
  Caster_Wheel_N°1/2(alpha1) -> alpha1/1  "alpha1"
  Demux/3 -> [Thetad_3]
  [Delta5] -> Caster_Wheel_N°5/4(Delta5)
  Demux1/1 -> [v_ruota1]
  Driving_Wheel_N°3/2(alpha3) -> alpha3/1  "alpha3"
  Demux1/6 -> [v_ruota6]
  Caster_Wheel_N°5/2(alpha5) -> alpha5/1  "alpha5"
  Demux1/2 -> [v_ruota2]
  Demux/1 -> [Thetad_1]
  Demux3/2 -> [Delta2]
  [v_ruota6] -> Caster_Wheel_N°6/2(vx_ruota6)
  Driving_Wheel_N°4/1(Sigma4) -> Sigma4/1  "Sigma4"
  Demux2/5 -> [gamma5]
  Caster_Wheel_N°6/2(alpha6) -> alpha6/1  "alpha2"
  Driving_Wheel_N°3/1(Sigma3) -> Sigma3/1  "Sigma3"
  [Thetad_1] -> Caster_Wheel_N°1/1(Thetad_1)
  Demux/2 -> [Thetad_2]
  Driving_Wheel_N°4/2(alpha4) -> alpha4/1  "alpha4"
  Demux1/4 -> [v_ruota4]
  Thetad_ruote/1 -> Demux/1
  [gamma6] -> Caster_Wheel_N°6/3(gamma6)
  Caster_Wheel_N°2/2(alpha2) -> alpha2/1  "alpha2"
  Caster_Wheel_N°5/1(Sigma5) -> Sigma5/1  "Sigma5"
  [v_ruota3] -> Driving_Wheel_N°3/2(vx_ruota3)
  Caster_Wheel_N°1/1(Sigma1) -> Sigma1/1  "Sigma1"
  [Thetad_4] -> Driving_Wheel_N°4/1(Thetad_4)
  Demux/5 -> [Thetad_5]
  Caster_Wheel_N°2/1(Sigma2) -> Sigma2/1  "Sigma2"
  [gamma1] -> Caster_Wheel_N°1/3(gamma1)
  Demux/4 -> [Thetad_4]
  [v_ruota4] -> Driving_Wheel_N°4/2(vx_ruota4)
  Demux3/1 -> [Delta1]
  Caster_Wheel_N°6/1(Sigma6) -> Sigma6/1  "Sigma2"
  Demux3/3 -> [Delta5]
  Demux/6 -> [Thetad_6]
  Demux2/6 -> [gamma6]
  [Thetad_5] -> Caster_Wheel_N°5/1(Thetad_5)
  [Delta1] -> Caster_Wheel_N°1/4(Delta1)
  Demux1/5 -> [v_ruota5]
  Delta/1 -> Demux3/1
  gamma/1 -> Demux2/1
  [Thetad_3] -> Driving_Wheel_N°3/1(Thetad_3)
  vx_ruote/1 -> Demux1/1
  Demux2/4 -> [gamma4]
  Demux2/1 -> [gamma1]
  Demux2/2 -> [gamma2]
  [v_ruota2] -> Caster_Wheel_N°2/2(vx_ruota2)
  [gamma5] -> Caster_Wheel_N°5/3(gamma5)
  Demux2/3 -> [gamma3]
  [gamma4] -> Driving_Wheel_N°4/3(gamma4)
  [Thetad_2] -> Caster_Wheel_N°2/1(Thetad_2)
  [v_ruota1] -> Caster_Wheel_N°1/2(vx_ruota1)
  [gamma2] -> Caster_Wheel_N°2/3(gamma2)
  Demux1/3 -> [v_ruota3]
  [Delta6] -> Caster_Wheel_N°6/4(Delta6)
  [Thetad_6] -> Caster_Wheel_N°6/1(Thetad_6)
  Demux3/4 -> [Delta6]
  [Delta2] -> Caster_Wheel_N°2/4(Delta2)
  [gamma3] -> Driving_Wheel_N°3/3(gamma3)
  [v_ruota5] -> Caster_Wheel_N°5/2(vx_ruota5)

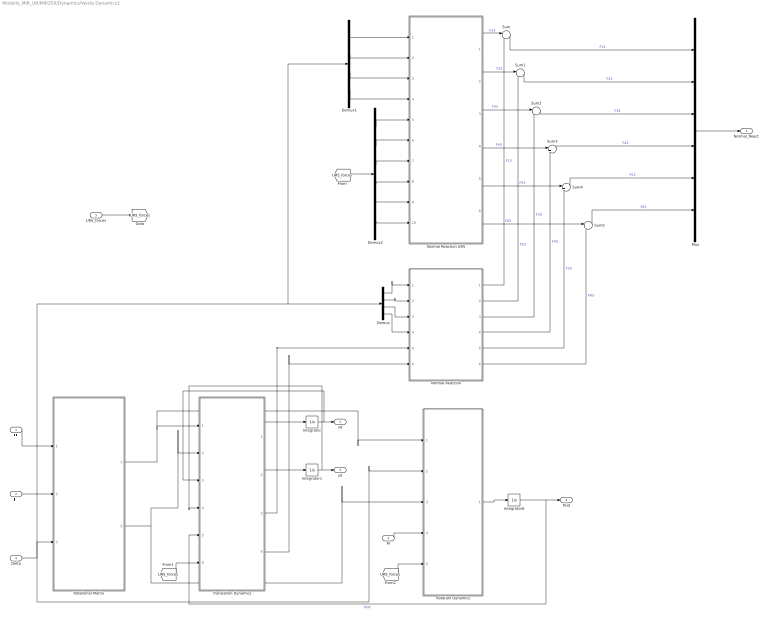
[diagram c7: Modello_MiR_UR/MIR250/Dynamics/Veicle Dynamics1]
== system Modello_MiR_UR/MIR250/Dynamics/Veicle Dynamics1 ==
  FL : Inport
  FT : Inport  Port=2
  M : Inport  Port=3
  Delta : Inport  Port=4
  UR5_forces : Inport  Port=5
  Demux : Demux
  Demux1 : Demux
  Demux2 : Demux  Outputs=6
  Integrator : Integrator
  Integrator1 : Integrator
  Integrator6 : Integrator
  Mux : Mux  Inputs=6
  Normal Reaction : Subsystem
  Normal Reaction UR5 : Subsystem
  Rotation Dynamics : Subsystem
  Rotational Matrix : MATLAB Function  TreatAsAtomicUnit=on
  Sum{,1..5} (6 alike) : Sum  Inputs=|++
  Translation Dynamics : Subsystem
  Normal_React : Outport
  xd : Outport  Port=2  PortDimensions=1
  yd : Outport  Port=3  PortDimensions=1
  Psid : Outport  Port=4  PortDimensions=1
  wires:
  Normal Reaction/4(F43) -> Sum3/2  "F43"
  Demux/1 -> Normal Reaction/1(Delta1)
  Demux/2 -> Normal Reaction/2(Delta2)
  Normal Reaction/5(F53) -> Sum4/2  "F53"
  Demux/4 -> Normal Reaction/4(Delta6)
  Normal Reaction/1(F13) -> Sum/2  "F13"
  Rotation Dynamics/1(Psidd) -> Integrator6/1
  Normal Reaction/2(F23) -> Sum1/2  "F23"
  Normal Reaction/6(F63) -> Sum5/2  "F63"
  Demux/3 -> Normal Reaction/3(Delta5)
  Normal Reaction/3(F33) -> Sum2/2  "F33"
  Integrator6/1 -> Psid/1, Translation Dynamics/5(Psid)  "Psid"
  Delta/1 -> Rotation Dynamics/2("Delta "), Demux1/1, Demux/1, Rotational Matrix/3(Delta)
  Rotational Matrix/2(Fy_generalized) -> Rotation Dynamics/3(Fy_generalized), Translation Dynamics/2(Fy_generalized)
  FL/1 -> Rotational Matrix/1(FL)
  FT/1 -> Rotational Matrix/2(FT)
  Rotational Matrix/1(Fx_generalized) -> Rotation Dynamics/1(Fx_generalized), Translation Dynamics/1(Fx_generalized)
  Translation Dynamics/1(xdd) -> Integrator/1
  Translation Dynamics/2(ydd) -> Integrator1/1
  Integrator/1 -> Translation Dynamics/3(xd), xd/1
  Integrator1/1 -> Translation Dynamics/4(yd), yd/1
  M/1 -> Rotation Dynamics/4(M)
  Translation Dynamics/3(a_tau) -> Normal Reaction/5(a_tau)
  Translation Dynamics/4(a_n) -> Normal Reaction/6(a_n)
  Demux1/3 -> Normal Reaction UR5/3(Delta5)
  Demux1/1 -> Normal Reaction UR5/1(Delta1)
  Demux1/2 -> Normal Reaction UR5/2(Delta2)
  Demux1/4 -> Normal Reaction UR5/4(Delta6)
  Demux2/1 -> Normal Reaction UR5/5(Rx)
  Demux2/2 -> Normal Reaction UR5/6(Ry)
  Demux2/3 -> Normal Reaction UR5/7(Rz)
  Demux2/4 -> Normal Reaction UR5/8(MRx)
  Demux2/5 -> Normal Reaction UR5/9(MRy)
  Demux2/6 -> Normal Reaction UR5/10(MRz)
  Normal Reaction UR5/1(F13) -> Sum/1  "F13"
  Sum/1 -> Mux/1  "F13"
  Normal Reaction UR5/2(F23) -> Sum1/1  "F23"
  Sum1/1 -> Mux/2  "F23"
  Normal Reaction UR5/3(F33) -> Sum2/1  "F33"
  Sum2/1 -> Mux/3  "F33"
  Normal Reaction UR5/4(F43) -> Sum3/1  "F43"
  Sum3/1 -> Mux/4  "F43"
  Normal Reaction UR5/5(F53) -> Sum4/1  "F53"
  Sum4/1 -> Mux/5  "F53"
  Normal Reaction UR5/6(F63) -> Sum5/1  "F63"
  Sum5/1 -> Mux/6  "F63"
  Mux/1 -> Normal_React/1
  UR5_forces/1 -> [UR5_forces]
  [UR5_forces] -> Demux2/1
  [UR5_forces] -> Translation Dynamics/6(UR5_forces)
  [UR5_forces] -> Rotation Dynamics/5(UR5_forces)

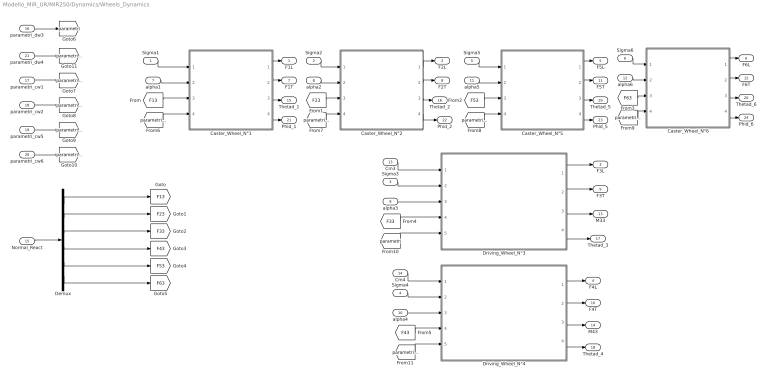
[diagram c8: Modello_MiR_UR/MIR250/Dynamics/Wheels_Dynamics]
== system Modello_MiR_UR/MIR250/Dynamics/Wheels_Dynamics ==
  Sigma1 : Inport
  Sigma2 : Inport  Port=2
  Sigma3 : Inport  Port=3
  Sigma4 : Inport  Port=4
  Sigma5 : Inport  Port=5
  Sigma6 : Inport  Port=6
  alpha1 : Inport  Port=7
  alpha2 : Inport  Port=8
  alpha3 : Inport  Port=9
  alpha4 : Inport  Port=10
  alpha5 : Inport  Port=11
  alpha6 : Inport  Port=12
  Cm3 : Inport  Port=13
  Cm4 : Inport  Port=14
  Normal_React : Inport  Port=15
  parametri_dw3 : Inport  Port=16
  parametri_cw1 : Inport  Port=17
  parametri_cw2 : Inport  Port=18
  parametri_cw5 : Inport  Port=19
  parametri_cw6 : Inport  Port=20
  parametri_dw4 : Inport  Port=21
  Caster_Wheel_N°1 : Subsystem
  Caster_Wheel_N°2 : Subsystem
  Caster_Wheel_N°5 : Subsystem
  Caster_Wheel_N°6 : Subsystem
  Demux : Demux  Outputs=6
  Driving_Wheel_N°3 : Subsystem
  Driving_Wheel_N°4 : Subsystem
  F1L : Outport
  F2L : Outport  Port=2
  F3L : Outport  Port=3
  F4L : Outport  Port=4
  F5L : Outport  Port=5
  F6L : Outport  Port=6
  F1T : Outport  Port=7
  F2T : Outport  Port=8
  F3T : Outport  Port=9
  F4T : Outport  Port=10
  F5T : Outport  Port=11
  F6T : Outport  Port=12
  M33 : Outport  Port=13
  M43 : Outport  Port=14
  Thetad_1 : Outport  Port=15
  Thetad_2 : Outport  Port=16
  Thetad_3 : Outport  Port=17
  Thetad_4 : Outport  Port=18
  Thetad_5 : Outport  Port=19
  Thetad_6 : Outport  Port=20
  Phid_1 : Outport  Port=21  PortDimensions=1
  Phid_2 : Outport  Port=22  PortDimensions=1
  Phid_5 : Outport  Port=23  PortDimensions=1
  Phid_6 : Outport  Port=24  PortDimensions=1
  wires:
  Sigma5/1 -> Caster_Wheel_N°5/1(Sigma5)
  Caster_Wheel_N°6/1(F6L) -> F6L/1
  Sigma2/1 -> Caster_Wheel_N°2/1(Sigma2)
  Caster_Wheel_N°6/3(Thetad_6) -> Thetad_6/1
  Caster_Wheel_N°2/1(F2L) -> F2L/1
  Caster_Wheel_N°6/4(Phid_6) -> Phid_6/1
  Caster_Wheel_N°5/3(Thetad_5) -> Thetad_5/1
  alpha1/1 -> Caster_Wheel_N°1/2(alpha1)
  Sigma1/1 -> Caster_Wheel_N°1/1(Sigma1)
  Caster_Wheel_N°1/2(F1T) -> F1T/1
  Caster_Wheel_N°1/4(Phid_1) -> Phid_1/1
  Caster_Wheel_N°5/2(F5T) -> F5T/1
  Caster_Wheel_N°5/4(Phid_5) -> Phid_5/1
  Caster_Wheel_N°5/1(F5L) -> F5L/1
  Caster_Wheel_N°6/2(F6T) -> F6T/1
  Sigma6/1 -> Caster_Wheel_N°6/1(Sigma6)
  alpha6/1 -> Caster_Wheel_N°6/2(alpha6)
  Caster_Wheel_N°2/4(Phid_2) -> Phid_2/1
  alpha5/1 -> Caster_Wheel_N°5/2(alpha5)
  Caster_Wheel_N°2/2(F2T) -> F2T/1
  Caster_Wheel_N°1/1(F1L) -> F1L/1
  alpha2/1 -> Caster_Wheel_N°2/2(alpha2)
  Caster_Wheel_N°2/3(Thetad_2) -> Thetad_2/1
  Caster_Wheel_N°1/3(Thetad_1) -> Thetad_1/1
  alpha4/1 -> Driving_Wheel_N°4/3(alpha4)
  alpha3/1 -> Driving_Wheel_N°3/3(alpha3)
  Driving_Wheel_N°4/2(F4T) -> F4T/1
  Driving_Wheel_N°3/3(M33) -> M33/1
  Driving_Wheel_N°4/4(Thetad_4) -> Thetad_4/1
  Sigma4/1 -> Driving_Wheel_N°4/2(Sigma4)
  Driving_Wheel_N°4/3(M43) -> M43/1
  Sigma3/1 -> Driving_Wheel_N°3/2(Sigma3)
  Driving_Wheel_N°3/1(F3L) -> F3L/1
  Cm3/1 -> Driving_Wheel_N°3/1(Cm3)
  Driving_Wheel_N°3/4(Thetad_3) -> Thetad_3/1
  Driving_Wheel_N°3/2(F3T) -> F3T/1
  Driving_Wheel_N°4/1(F4L) -> F4L/1
  Cm4/1 -> Driving_Wheel_N°4/1(Cm4)
  Normal_React/1 -> Demux/1
  [F13] -> Caster_Wheel_N°1/3(F13)
  [F23] -> Caster_Wheel_N°2/3(F23)
  [F53] -> Caster_Wheel_N°5/3(F53)
  [F63] -> Caster_Wheel_N°6/3(F63)
  [F33] -> Driving_Wheel_N°3/4(F33)
  [F43] -> Driving_Wheel_N°4/4(F43)
  Demux/1 -> [F13]
  Demux/2 -> [F23]
  Demux/3 -> [F33]
  Demux/4 -> [F43]
  Demux/5 -> [F53]
  Demux/6 -> [F63]
  parametri_dw3/1 -> [parametri]
  [parametri_cw1] -> Caster_Wheel_N°1/4(parametri_cw1)
  [parametri_cw2] -> Caster_Wheel_N°2/4(parametri)
  [parametri_cw5] -> Caster_Wheel_N°5/4(parametri)
  [parametri_cw6] -> Caster_Wheel_N°6/4(parametri)
  [parametri] -> Driving_Wheel_N°3/5(parametri_dw3)
  [parametri_dw4] -> Driving_Wheel_N°4/5(parametri_dw4)
  parametri_cw1/1 -> [parametri_cw1]
  parametri_cw2/1 -> [parametri_cw2]
  parametri_cw5/1 -> [parametri_cw5]
  parametri_cw6/1 -> [parametri_cw6]
  parametri_dw4/1 -> [parametri_dw4]
